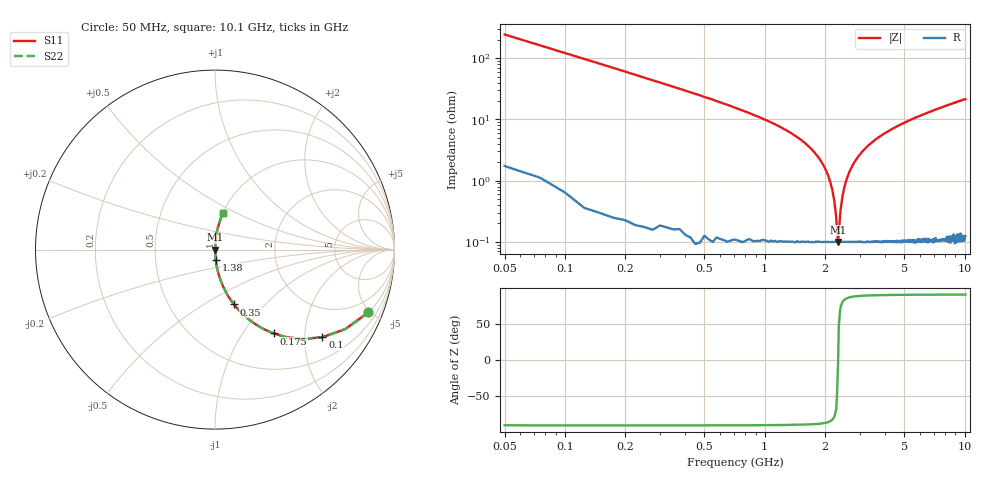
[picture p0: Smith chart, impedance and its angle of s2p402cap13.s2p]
! AVX Thin Film Operation		Date: April 2003
! Description: Accu-P® Series, Thin Film, SMD, RF Capacitor
! Part Number: 04023K130FBS
! 50 MHz  -  10.05 GHz
! Serial Measurements
# hz S db R 50
!	S11		S21		S12		S22
!	dB	Phase	dB	Phase	dB	Phase	dB	Phase
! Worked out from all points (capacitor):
!   400 points, 50 MHz to 10.1 GHz, reference 50 ohm
!   read as one part in series: C = 13 pF near 100 MHz
!   lowest |Z| = 100 mohm at 2.33 GHz (marker M1)
!   series resonance near 2.331 GHz, so ESL is about 360 pH
!   S11 on the Smith chart (normalised r, x): 50 MHz: 1.04, -4.88; 100 MHz: 1.01, -2.44; 175 MHz: 1.01, -1.39; 350 MHz: 1.00, -0.68; 1.38 GHz: 1.00, -0.12; 10.1 GHz: 1.00, +0.43
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5e7  -0.70 -22.2  -8.47 67.4  -8.47 67.4  -0.70 -22.2
1e8  -2.25 -39.2  -3.99 50.5  -3.99 50.5  -2.25 -39.2
1.75e8  -4.88 -55.0  -1.73 34.8  -1.73 34.8  -4.88 -55.0
3.5e8  -9.81 -70.9  -0.49 18.8  -0.49 18.8  -9.81 -70.9
7e8  -16.10 -80.6  -0.12 9.0  -0.12 9.0  -16.10 -80.6
1.38e9  -24.80 -85.7  -0.02 3.3  -0.02 3.3  -24.80 -85.7
1.73e9  -29.90 -86.4  -0.01 1.8  -0.01 1.8  -29.90 -86.4
1.98e9  -35.20 -85.7  -0.01 1.0  -0.01 1.0  -35.20 -85.7
2.18e9  -42.90 -81.6  -0.01 0.4  -0.01 0.4  -42.90 -81.6
2.23e9  -46.40 -77.7  -0.01 0.3  -0.01 0.3  -46.40 -77.7
2.28e9  -51.80 -66.9  -0.01 0.1  -0.01 0.1  -51.80 -66.9
2.3e9  -56.10 -50.2  -0.01 0.1  -0.01 0.1  -56.10 -50.2
2.33e9  -60.00 -3.8  -0.01 0.0  -0.01 0.0  -60.00 -3.8
2.4e9  -49.30 72.8  -0.01 -0.2  -0.01 -0.2  -49.30 72.8
2.45e9  -45.10 79.3  -0.01 -0.3  -0.01 -0.3  -45.10 79.3
2.6e9  -38.60 84.5  -0.01 -0.7  -0.01 -0.7  -38.60 84.5
2.9e9  -32.60 86.2  -0.01 -1.3  -0.01 -1.3  -32.60 86.2
3.4e9  -27.80 86.3  -0.02 -2.3  -0.02 -2.3  -27.80 86.3
5.08e9  -20.90 84.2  -0.04 -5.2  -0.04 -5.2  -20.90 84.2
6.75e9  -17.50 81.9  -0.09 -7.7  -0.09 -7.7  -17.50 81.9
8.43e9  -15.20 79.7  -0.14 -10.0  -0.14 -10.0  -15.20 79.7
1.01e10  -13.60 77.6  -0.21 -12.1  -0.21 -12.1  -13.60 77.6
